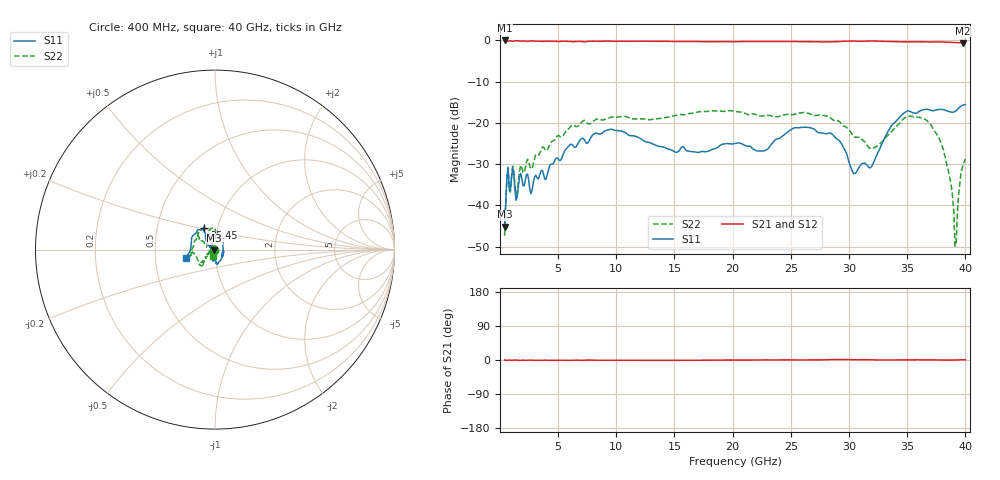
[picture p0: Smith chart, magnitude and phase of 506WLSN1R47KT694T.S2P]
!  American Technical Ceramics  Date:  8/31/2012
!  One Norden Lane
!  Huntington Station,  NY.  11746-2102
!  Tel:  (631) 622-4700  Fax:  (631) 622-4748
!  Part Number  506WLSN1R47KG694T
!  Description:  Ultra-Broadband Inductor
!  Application:  Ultra-broadband DC block decoupling, bias tee
# GHZ S DB R 50
! Freq  |S11|  S11 Ph  |S21|  S21 Ph  |S12|  S12 Ph  |S22|  S22 Ph
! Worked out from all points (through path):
!   401 points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, 400 MHz to 40 GHz, reference 50 ohm
!   highest |S21| = -0.01 dB at 400 MHz (marker M1); lowest = -0.6 dB at 39.8 GHz (marker M2)
!   lowest |S11| = -45.2 dB at 400 MHz (marker M3), VSWR 1.01, Z = 49.6 - j0.341 ohm
!   |S11| at or under -10 dB: start of sweep to end of sweep
!   |S22| runs from -49.9 to -17.0 dB; largest |S21 - S12| = 0.0023
!   S11 on the Smith chart (normalised r, x): 400 MHz: 0.99, -0.01; 35.45 GHz: 0.86, +0.21; 40 GHz: 0.72, -0.07
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0.4  -45.16 -141.4  -0.01 -0.2  -0.01 -0.2  -47.32 -131.5
0.895  -36.36 -150.5  -0.09 -0.5  -0.09 -0.5  -36.76 -149.1
1.489  -37.78 -143.9  -0.07 -0.5  -0.08 -0.5  -36.52 -147.2
2.677  -37.18 -141.1  -0.13 -0.4  -0.14 -0.4  -31.16 -158.1
7.033  -23.74 -97.1  -0.27 -0.9  -0.26 -0.8  -19.75 -131.9
9.607  -21.51 -81.5  -0.18 -0.8  -0.18 -0.8  -18.59 -129.1
13.666  -25.68 -34.0  -0.22 -1.0  -0.22 -0.9  -18.93 -163.1
20.2  -24.96 -39.7  -0.28 -0.0  -0.28 0.0  -17.19 -168.2
22.675  -26.75 12.5  -0.27 0.2  -0.26 0.2  -18.29 169.4
26.833  -21.30 90.8  -0.28 0.2  -0.28 0.2  -17.98 135.1
29.11  -24.14 114.8  -0.29 1.5  -0.29 1.5  -19.53 145.5
30.496  -32.25 145.1  -0.17 0.7  -0.17 0.7  -23.45 150.8
31.981  -30.38 146.7  -0.14 0.4  -0.14 0.4  -26.05 147.9
33.466  -21.49 128.6  -0.26 0.0  -0.26 0.0  -22.57 125.0
35.446  -17.50 116.6  -0.35 0.4  -0.36 0.4  -18.38 93.7
36.733  -16.69 132.4  -0.36 0.2  -0.38 0.2  -19.53 87.7
37.921  -16.74 151.2  -0.35 -0.0  -0.36 -0.1  -24.96 87.4
38.713  -17.34 167.6  -0.46 -0.1  -0.47 -0.1  -34.16 102.2
39.109  -17.20 -179.2  -0.52 0.0  -0.53 0.1  -49.86 122.4
39.307  -16.79 -173.0  -0.53 0.1  -0.54 0.3  -42.10 -103.8
39.802  -15.65 -166.3  -0.60 0.5  -0.61 0.6  -30.12 -104.5
40  -15.54 -164.1  -0.59 0.9  -0.60 0.9  -28.74 -104.3
